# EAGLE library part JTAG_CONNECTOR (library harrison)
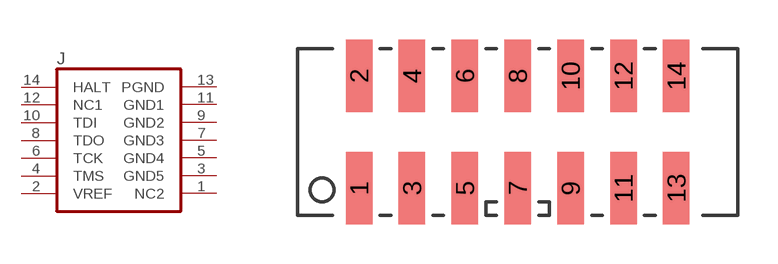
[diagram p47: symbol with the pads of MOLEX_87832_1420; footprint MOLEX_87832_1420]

Designator prefix J

## JTAG_CONNECTOR  [MOLEX_87832_1420]
1  NC2  nc
2  VREF  in
3  GND5  nc
4  TMS  in
5  GND4  nc
6  TCK  in
7  GND3  nc
8  TDO  in
9  GND2  nc
10  TDI  in
11  GND1  nc
12  NC1  pwr
13  PGND  pwr
14  HALT  pwr

## Footprint MOLEX_87832_1420 (pad centres in mm)
smd 1 x 2.75: 1 -6,-2.125; 2 -6,2.125; 3 -4,-2.125; 4 -4,2.125; 5 -2,-2.125; 6 -2,2.125; 7 0,-2.125; 8 0,2.125; 9 2,-2.125; 10 2,2.125; 11 4,-2.125; 12 4,2.125; 13 6,-2.125; 14 6,2.125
